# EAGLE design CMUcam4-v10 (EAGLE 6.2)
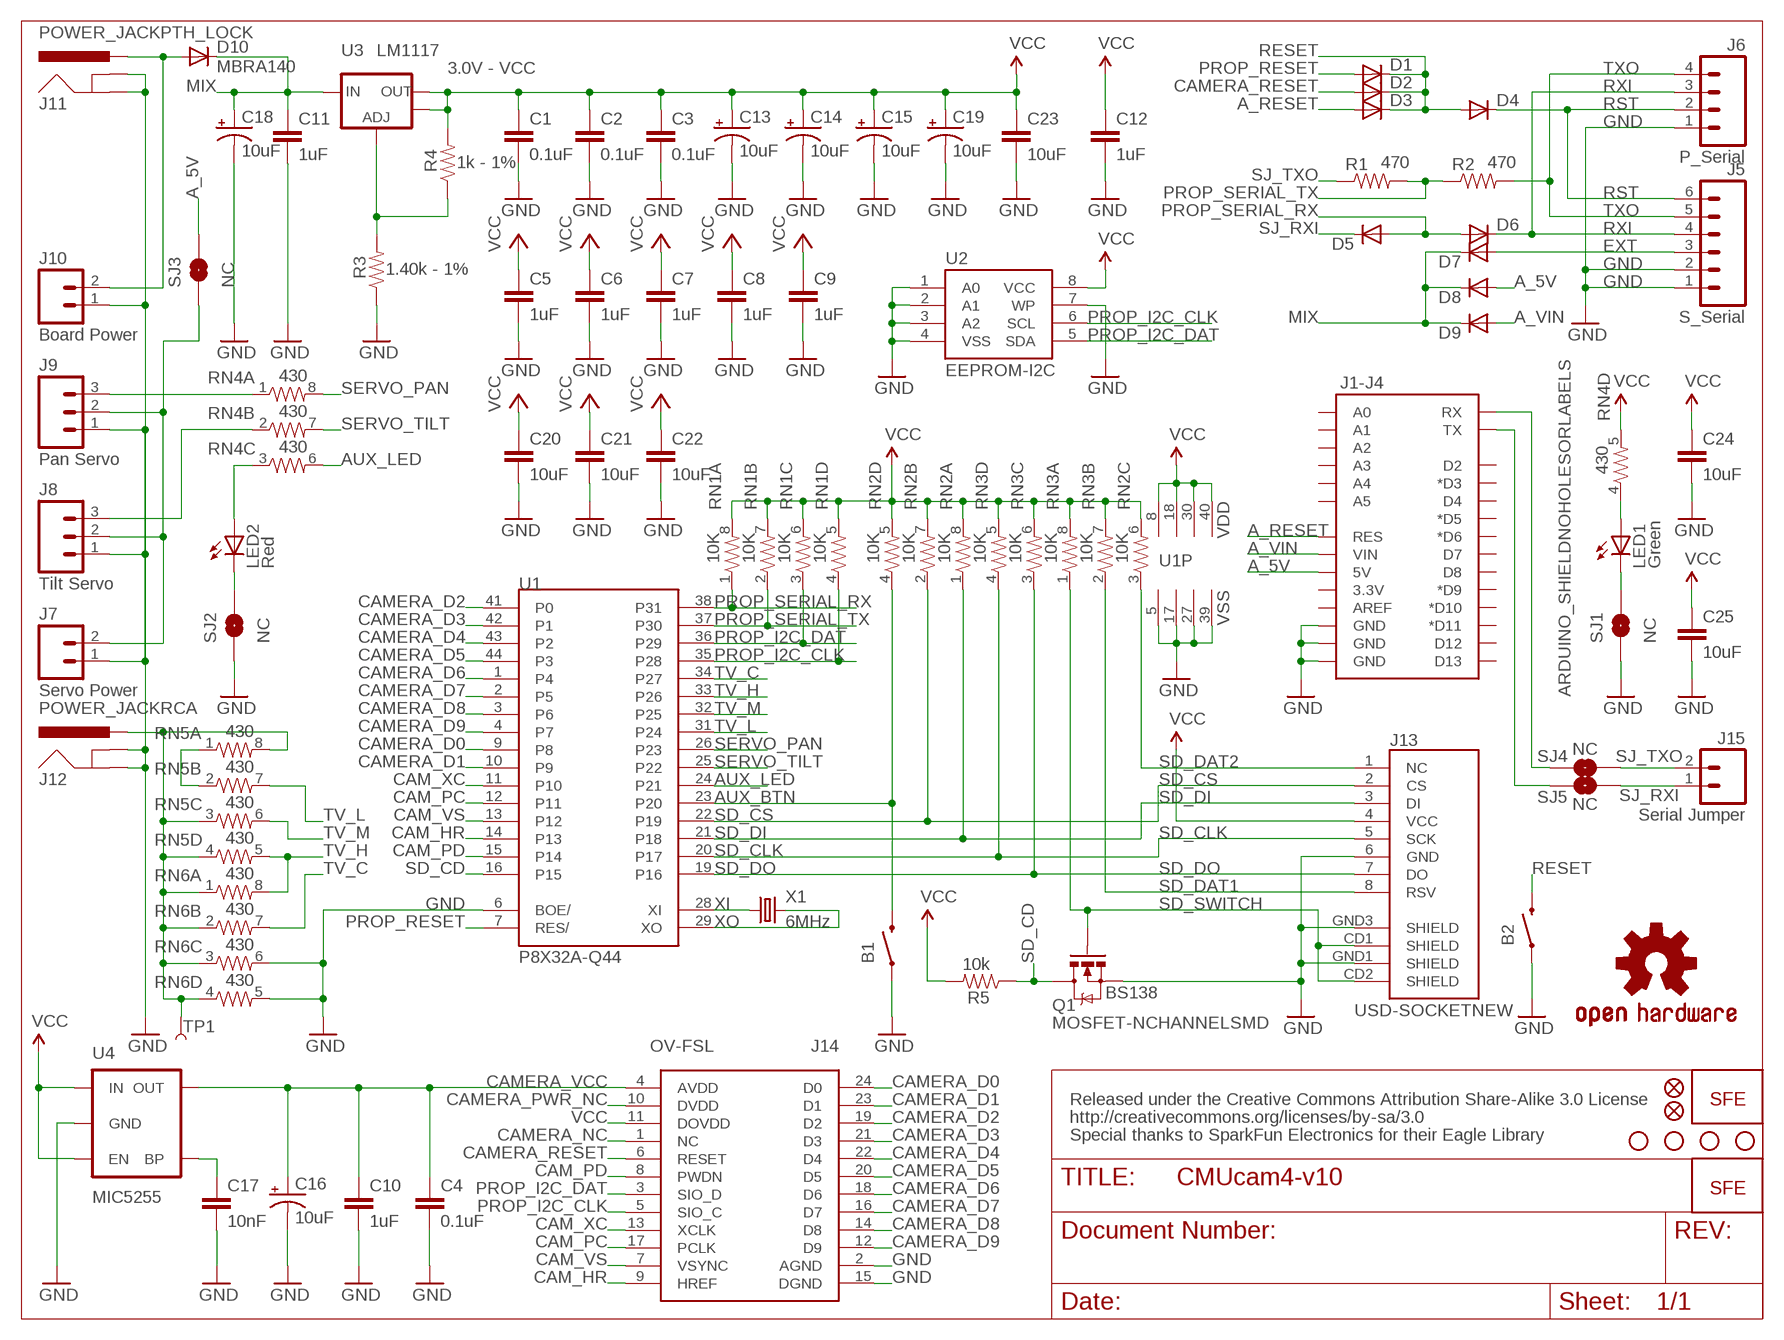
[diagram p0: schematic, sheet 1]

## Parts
B1  SWITCH-MOMENTARY-2SMD  [TACTILE_SWITCH_SMD]
B2  SWITCH-MOMENTARY-2SMD  [TACTILE_SWITCH_SMD]
C1  0.1uF  CAP0402-CAP  [0402-CAP]
C2  0.1uF  CAP0402-CAP  [0402-CAP]
C3  0.1uF  CAP0402-CAP  [0402-CAP]
C4  0.1uF  CAP0402-CAP  [0402-CAP]
C5  1uF  CAP0402-CAP  [0402-CAP]
C6  1uF  CAP0402-CAP  [0402-CAP]
C7  1uF  CAP0402-CAP  [0402-CAP]
C8  1uF  CAP0402-CAP  [0402-CAP]
C9  1uF  CAP0402-CAP  [0402-CAP]
C10  1uF  CAP0402-CAP  [0402-CAP]
C11  1uF  CAP0402-CAP  [0402-CAP]
C12  1uF  CAP0402-CAP  [0402-CAP]
C13  10uF  CAP_POL1206  [EIA3216]
C14  10uF  CAP_POL1206  [EIA3216]
C15  10uF  CAP_POL1206  [EIA3216]
C16  10uF  CAP_POL1206  [EIA3216]
C17  10nF  CAP0402-CAP  [0402-CAP]
C18  10uF  CAP_POL1206  [EIA3216]
C19  10uF  CAP_POL1206  [EIA3216]
C20  10uF  CAP0402-CAP  [0402-CAP]
C21  10uF  CAP0402-CAP  [0402-CAP]
C22  10uF  CAP0402-CAP  [0402-CAP]
C23  10uF  CAP0402-CAP  [0402-CAP]
C24  10uF  CAP0402-CAP  [0402-CAP]
C25  10uF  CAP0402-CAP  [0402-CAP]
D1  DIODESOD523  [SOD523]
D2  DIODESOD523  [SOD523]
D3  DIODESOD523  [SOD523]
D4  DIODESOD523  [SOD523]
D5  DIODESOD523  [SOD523]
D6  DIODESOD523  [SOD523]
D7  DIODESMA  [SMA-DIODE]
D8  DIODESMA  [SMA-DIODE]
D9  DIODESMA  [SMA-DIODE]
D10  MBRA140  DIODESMA  [SMA-DIODE]
J1-J4  ARDUINO_SHIELDNOHOLESORLABELS  [DUEMILANOVE_SHIELD_NOHOLES_NOLABELS]
J5  S_Serial  M06SIP  [1X06]
J6  P_Serial  M04PTH  [1X04]
J7  Servo Power  M02PTH  [1X02]
J8  Tilt Servo  M03PTH  [1X03]
J9  Pan Servo  M03PTH  [1X03]
J10  Board Power  M02PTH  [1X02]
J11  POWER_JACKPTH_LOCK  [POWER_JACK_PTH_LOCK]
J12  POWER_JACKRCA  [RCA]
J13  USD-SOCKETNEW  [MICRO-SD-SOCKET-PP]
J14  OV-FSL  [OV-FSL]
J15  Serial Jumper  M02PTH  [1X02]
JP1  LOGO-SFENEW  [SFE-NEW-WEBLOGO]
JP2  LOGO-SFESK  [SFE-LOGO-FLAME]
JP3  FIDUCIALUFIDUCIAL  [MICRO-FIDUCIAL]
JP4  FIDUCIALUFIDUCIAL  [MICRO-FIDUCIAL]
LED1  Green  LED0603  [LED-0603]
LED2  Red  LED0603  [LED-0603]
Q1  MOSFET-NCHANNELSMD  [SOT23-3]
R1  470  RESISTOR0402-RES  [0402-RES]
R2  470  RESISTOR0402-RES  [0402-RES]
R3  1.40k - 1%  RESISTOR0402-RES  [0402-RES]
R4  1k - 1%  RESISTOR0402-RES  [0402-RES]
R5  10k  RESISTOR0402-RES  [0402-RES]
RN1  10K  4R-N0603-ARV  [0603-ARV]
RN2  10K  4R-N0603-ARV  [0603-ARV]
RN3  10K  4R-N0603-ARV  [0603-ARV]
RN4  430  4R-N0603-ARV  [0603-ARV]
RN5  430  4R-N0603-ARV  [0603-ARV]
RN6  430  4R-N0603-ARV  [0603-ARV]
SJ1  NC  SOLDERJUMPERTRACE  [SJ_2S-TRACE]
SJ2  NC  SOLDERJUMPERTRACE  [SJ_2S-TRACE]
SJ3  NC  SOLDERJUMPERNO  [SJ_2S-NO]
SJ4  NC  SOLDERJUMPERTRACE  [SJ_2S-TRACE]
SJ5  NC  SOLDERJUMPERTRACE  [SJ_2S-TRACE]
STD1  STAND-OFF  [STAND-OFF]
STD2  STAND-OFF  [STAND-OFF]
STD3  STAND-OFF  [STAND-OFF]
STD4  STAND-OFF  [STAND-OFF]
TP1  TEST-POINT3  [PAD.03X.03]
U1  P8X32A-Q44  [P8X32A-Q44]
U2  EEPROM-I2C  [SO08-EIAJ]
U3  LM1117  V_REG_LM1117SOT223  [SOT223]
U4  MIC5255  V_REG_LDOSMD  [SOT23-5]
U$1  OSHW-LOGOM  [OSHW-LOGO-M]
X1  6MHz  CRYSTALHC49UP  [HC49UP]

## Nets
A_5V: D8.A J1-J4.5V SJ3.2
A_RESET: D3.A J1-J4.RES
A_VIN: D9.A J1-J4.VIN
ADJUST: R3.2 R4.1 U3.1(ADJ)
AUX_BTN: B1.3 RN2.4 U1.23(P20)
AUX_LED: RN4.6 U1.24(P21)
BYP: C17.1 U4.4(BP)
CAM_HR: J14.9(HREF) U1.14(P13)
CAM_PC: J14.17(PCLK) U1.12(P11)
CAM_PD: J14.8(PWDN) U1.15(P14)
CAM_VS: J14.7(VSYNC) U1.13(P12)
CAM_XC: J14.13(XCLK) U1.11(P10)
CAMERA_D0: J14.24(D0) U1.9(P8)
CAMERA_D1: J14.23(D1) U1.10(P9)
CAMERA_D2: J14.19(D2) U1.41(P0)
CAMERA_D3: J14.21(D3) U1.42(P1)
CAMERA_D4: J14.22(D4) U1.43(P2)
CAMERA_D5: J14.20(D5) U1.44(P3)
CAMERA_D6: J14.18(D6) U1.1(P4)
CAMERA_D7: J14.16(D7) U1.2(P5)
CAMERA_D8: J14.14(D8) U1.3(P6)
CAMERA_D9: J14.12(D9) U1.4(P7)
CAMERA_NC: J14.1(NC)
CAMERA_PWR_NC: J14.10(DVDD)
CAMERA_RESET: D2.A J14.6(RESET)
CAMERA_VCC: C4.1 C10.1 C16.A(+) J14.4(AVDD) U4.5(OUT)
D0_TXO: J1-J4.RX SJ4.1
D1_RXI: J1-J4.TX SJ5.1
EXT: D7.A J5.3
GND [vcc]: B1.1 B2.1 C1.2 C2.2 C3.2 C4.2 C5.2 C6.2 C7.2 C8.2 C9.2 C10.2 C11.2 C12.2 C13.C(-) C14.C(-) C15.C(-) C16.C(-) C17.2 C18.C(-) C19.C(-) C20.2 C21.2 C22.2 C23.2 C24.2 C25.2 J1-J4.GND@0(GND) J1-J4.GND@1(GND) J1-J4.GND@2(GND) J5.1 J5.2 J6.1 J7.1 J8.1 J9.1 J10.1 J11.GND J11.GNDBREAK J12.BARREL(GND) J12.SPRING(GNDBREAK) J13.6(GND) J13.GND1(SHIELD) J13.GND3(SHIELD) J14.2(AGND) J14.15(DGND) Q1.2(S) R3.1 RN6.5 RN6.6 SJ1.1 SJ2.1 U1.5(VSS) U1.6(BOE/) U1.17(VSS) U1.27(VSS) U1.39(VSS) U2.1(A0) U2.2(A1) U2.3(A2) U2.4(VSS) U2.7(WP) U4.2(GND)
GREEN_BRIDGE: LED1.C SJ1.2
GREEN_CTRL: LED1.A RN4.4
MIX: C11.1 C18.A(+) D7.C D8.C D9.C D10.C U3.3(IN)
PROP_I2C_CLK: J14.5(SIO_C) RN1.4 U1.35(P28) U2.6(SCL)
PROP_I2C_DAT: J14.3(SIO_D) RN1.3 U1.36(P29) U2.5(SDA)
PROP_RESET: D1.A U1.7(RES/)
PROP_SERIAL_RX: D5.A D6.A RN1.1 U1.38(P31)
PROP_SERIAL_TX: R1.2 R2.1 RN1.2 U1.37(P30)
RED_BRIDGE: LED2.C SJ2.2
RED_CTRL: LED2.A RN4.3
RESET: B2.3 D1.C D2.C D3.C D4.A
RST: D4.C J5.6 J6.2
RXI: D6.C J5.4 J6.3
SD_CD: Q1.3(D) R5.1 U1.16(P15)
SD_CLK: J13.5(SCK) RN3.4 U1.20(P17)
SD_CS: J13.2(CS) RN2.2 U1.22(P19)
SD_DAT1: J13.8(RSV) RN3.2
SD_DAT2: J13.1(NC) RN2.3
SD_DI: J13.3(DI) RN2.1 U1.21(P18)
SD_DO: J13.7(DO) RN3.3 U1.19(P16)
SD_SWITCH: J13.CD1(SHIELD) J13.CD2(SHIELD) Q1.1(G) RN3.1
SERVO_PAN: RN4.8 U1.26(P23)
SERVO_PAN_IO: J9.3 RN4.1
SERVO_PWR: J7.2 J8.2 J9.2 SJ3.1
SERVO_TILT: RN4.7 U1.25(P22)
SERVO_TILT_IO: J8.3 RN4.2
SJ_RXI: D5.C J15.1 SJ5.2
SJ_TXO: J15.2 R1.1 SJ4.2
SYSTEM_VIN: D10.A J10.2 J11.PWR
TV: J12.BREAK(PWR) RN5.3 RN5.4 RN5.8 RN6.1 RN6.2 RN6.3 RN6.4 TP1.P$1
TV_C: RN6.7 U1.34(P27)
TV_H: RN5.5 RN6.8 U1.33(P26)
TV_L: RN5.7 U1.31(P24)
TV_M: RN5.6 U1.32(P25)
TV_R: RN5.1 RN5.2
TXO: J5.5 J6.4 R2.2
VCC: C1.1 C2.1 C3.1 C5.1 C6.1 C7.1 C8.1 C9.1 C12.1 C13.A(+) C14.A(+) C15.A(+) C19.A(+) C20.1 C21.1 C22.1 C23.1 C24.1 C25.1 J13.4(VCC) J14.11(DOVDD) R4.2 R5.2 RN1.5 RN1.6 RN1.7 RN1.8 RN2.5 RN2.6 RN2.7 RN2.8 RN3.5 RN3.6 RN3.7 RN3.8 RN4.5 U1.8(VDD) U1.18(VDD) U1.30(VDD) U1.40(VDD) U2.8(VCC) U3.2(OUT) U3.4(OUT) U4.1(IN) U4.3(EN)
XI: U1.28(XI) X1.1
XO: U1.29(XO) X1.2
Unconnected: J1-J4.3.3V J1-J4.A0 J1-J4.A1 J1-J4.A2 J1-J4.A3 J1-J4.A4 J1-J4.A5 J1-J4.AREF J1-J4.D2 J1-J4.D3(*D3) J1-J4.D4 J1-J4.D5(*D5) J1-J4.D6(*D6) J1-J4.D7 J1-J4.D8 J1-J4.D9(*D9) J1-J4.D10(*D10) J1-J4.D11(*D11) J1-J4.D12 J1-J4.D13

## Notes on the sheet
- 3.0V - VCC
- BS138
- Released under the Creative Commons Attribution Share-Alike 3.0 License
- http://creativecommons.org/licenses/by-sa/3.0
- Special thanks to SparkFun Electronics for their Eagle Library

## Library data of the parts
B1 B2 = SparkFun:SWITCH-MOMENTARY-2
C1-C12 C17 C20-C25 = SparkFun:CAP: Capacitor
C13-C16 C18 C19 = SparkFun:CAP_POL: Capacitor Polarized
D1-D6 = SparkFun-DiscreteSemi:DIODE: Diode
D7-D10 = SparkFun:DIODE: Diode
J1-J4 = SparkFun:ARDUINO_SHIELD
J5 = SparkFun:M06: Header 6 Standard 6-pin 0.1" header. Use with straight break away headers (SKU : PRT-00116), right angle break away headers (PRT-00553), swiss pins (PRT-00743), machine pins (PRT-00117), and female headers (PRT-00115). Molex polarized connector foot print use with SKU : PRT-08094 with associated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
J6 = SparkFun:M04: Header 4 Standard 4-pin 0.1" header. Use with straight break away headers (SKU : PRT-00116), right angle break away headers (PRT-00553), swiss pins (PRT-00743), machine pins (PRT-00117), and female headers (PRT-00115). Molex polarized connector foot print use with SKU : PRT-08231 with associated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
J7 J10 J15 = SparkFun:M02: Header 2
J8 J9 = SparkFun:M03: Header 3 Standard 3-pin 0.1" header. Use with straight break away headers (SKU : PRT-00116), right angle break away headers (PRT-00553), swiss pins (PRT-00743), machine pins (PRT-00117), and female headers (PRT-00115). Molex polarized connector foot print use with SKU : PRT-08232 with associated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
J11 J12 = SparkFun:POWER_JACK: Power Jack This is the standard 5.5mm barrel jack for power. The PTH is the most common, proven, reliable, footprint. All others are experimental. The Slot footprint only works if the mill layer is transmitted to the PCB fab house so be warned. Spark Fun Electronics SKU : PRT-00119. Mating wall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
J13 = SparkFun:USD-SOCKET: microSD Socket Push-push type uSD socket. Schematic element and footprint production proven. Spark Fun Electronics SKU : PRT-00127. tDoc lines correctly indicate media card edge positions when inserting (unlocked, locked, depressed).
J14 = ovt-breakout:OV-FSL
JP1 JP2 = SparkFun:LOGO-SFE: Spark Fun Electronics PCB Logo
JP3 JP4 = SparkFun:FIDUCIAL: Fiducial Alignment Points
LED1 LED2 = SparkFun:LED: LEDs
Q1 = SparkFun:MOSFET-NCHANNEL
R1-R5 = SparkFun:RESISTOR: Resistor
RN1-RN6 = resistor-dil:4R-N: Array Chip Resistor Source: RS Component / Phycomp
SJ1-SJ5 = SparkFun:SOLDERJUMPER: Solder Jumper
STD1-STD4 = SparkFun:STAND-OFF: Stand Off
TP1 = SparkFun-Passives:TEST-POINT: Bare copper test points for troubleshooting or ICT
U1 = parallax-propeller:P8X32A-Q44
U2 = SparkFun:EEPROM-I2C
U3 = SparkFun:V_REG_LM1117: Voltage Regulator LM1117 Standard adjustable voltage regulator but in SMD form. Spark Fun Electronics SKU : COM-00595
U4 = SparkFun:V_REG_LDO: Voltage Regulator LDO Standard 150mA LDO voltage regulator in SOT-23 layout. Micrel part MIC5205. BP (by-pass) pin is used to lower output noise with 470pF cap.
U$1 = SparkFun:OSHW-LOGO: Open Source Hardware Logo This logo indicates the piece of hardware it is found on incorporates a OSHW license and/or adheres to the definition of open source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
X1 = crystal:CRYSTAL: CRYSTAL; OC_FARNELL: unknown; OC_NEWARK: unknown

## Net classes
0 default: width 0.203 mm
1 vcc: width 0.254 mm

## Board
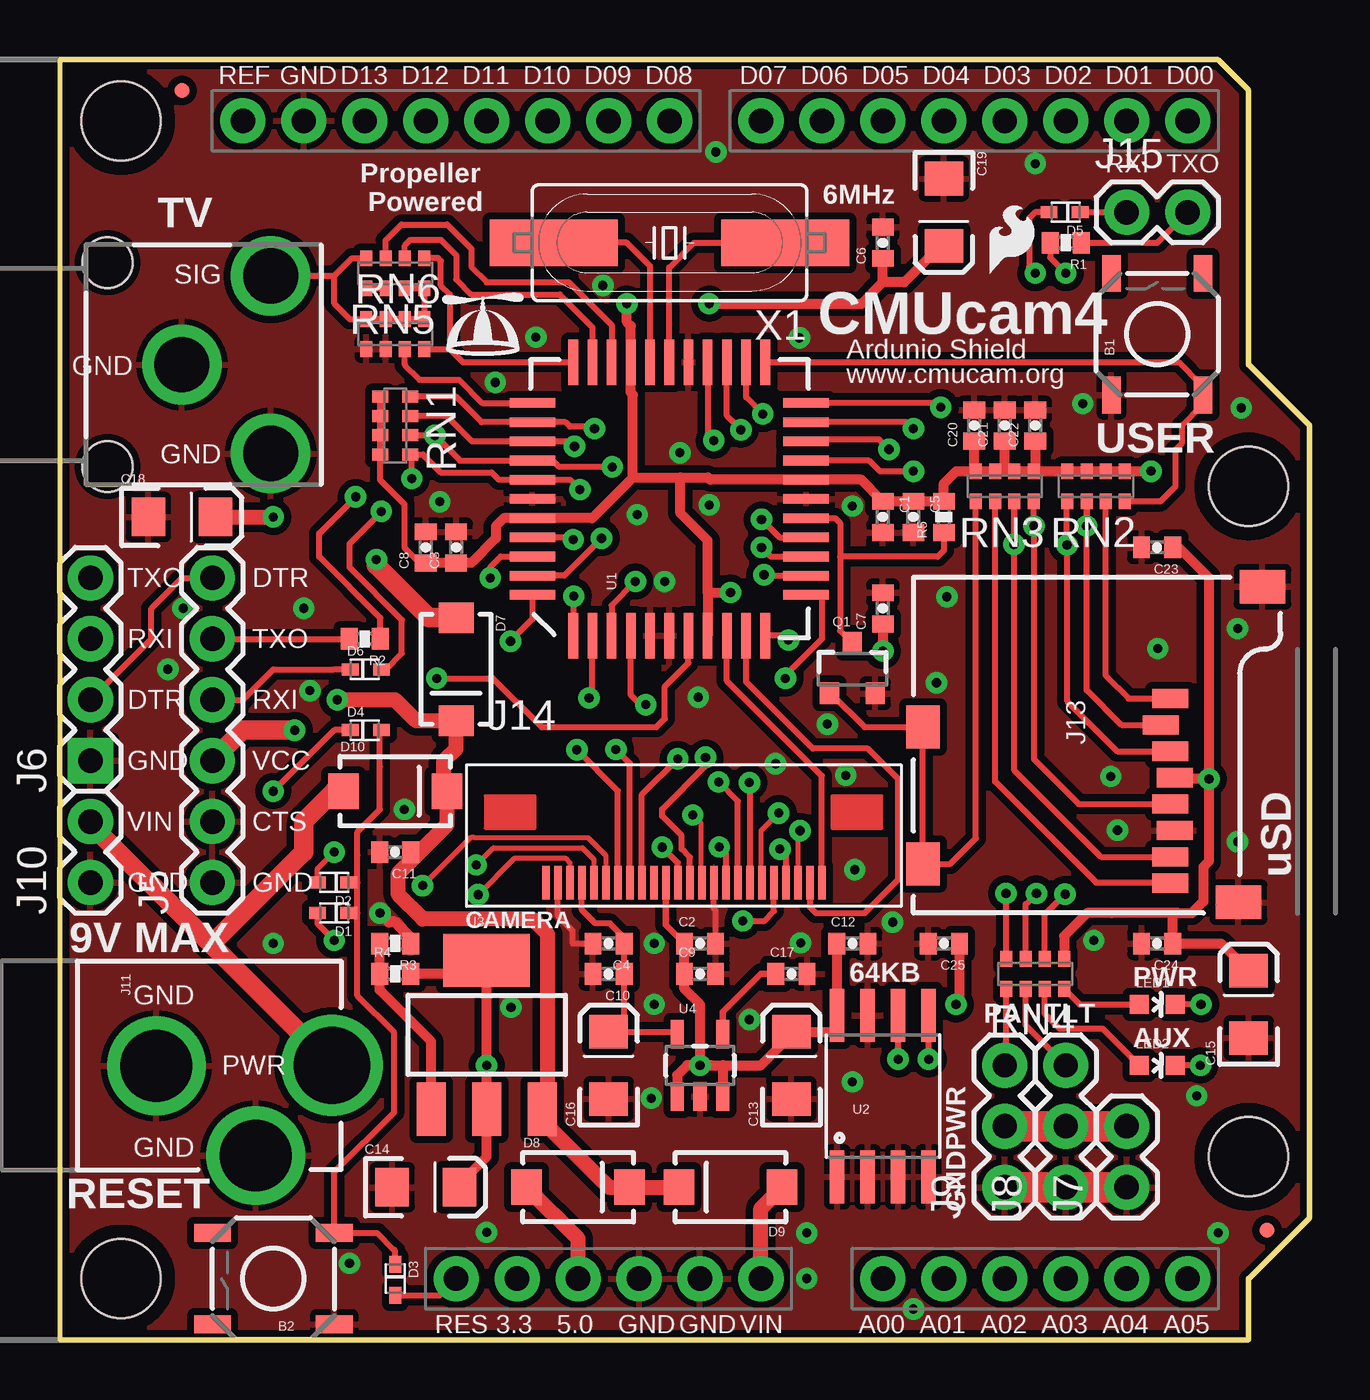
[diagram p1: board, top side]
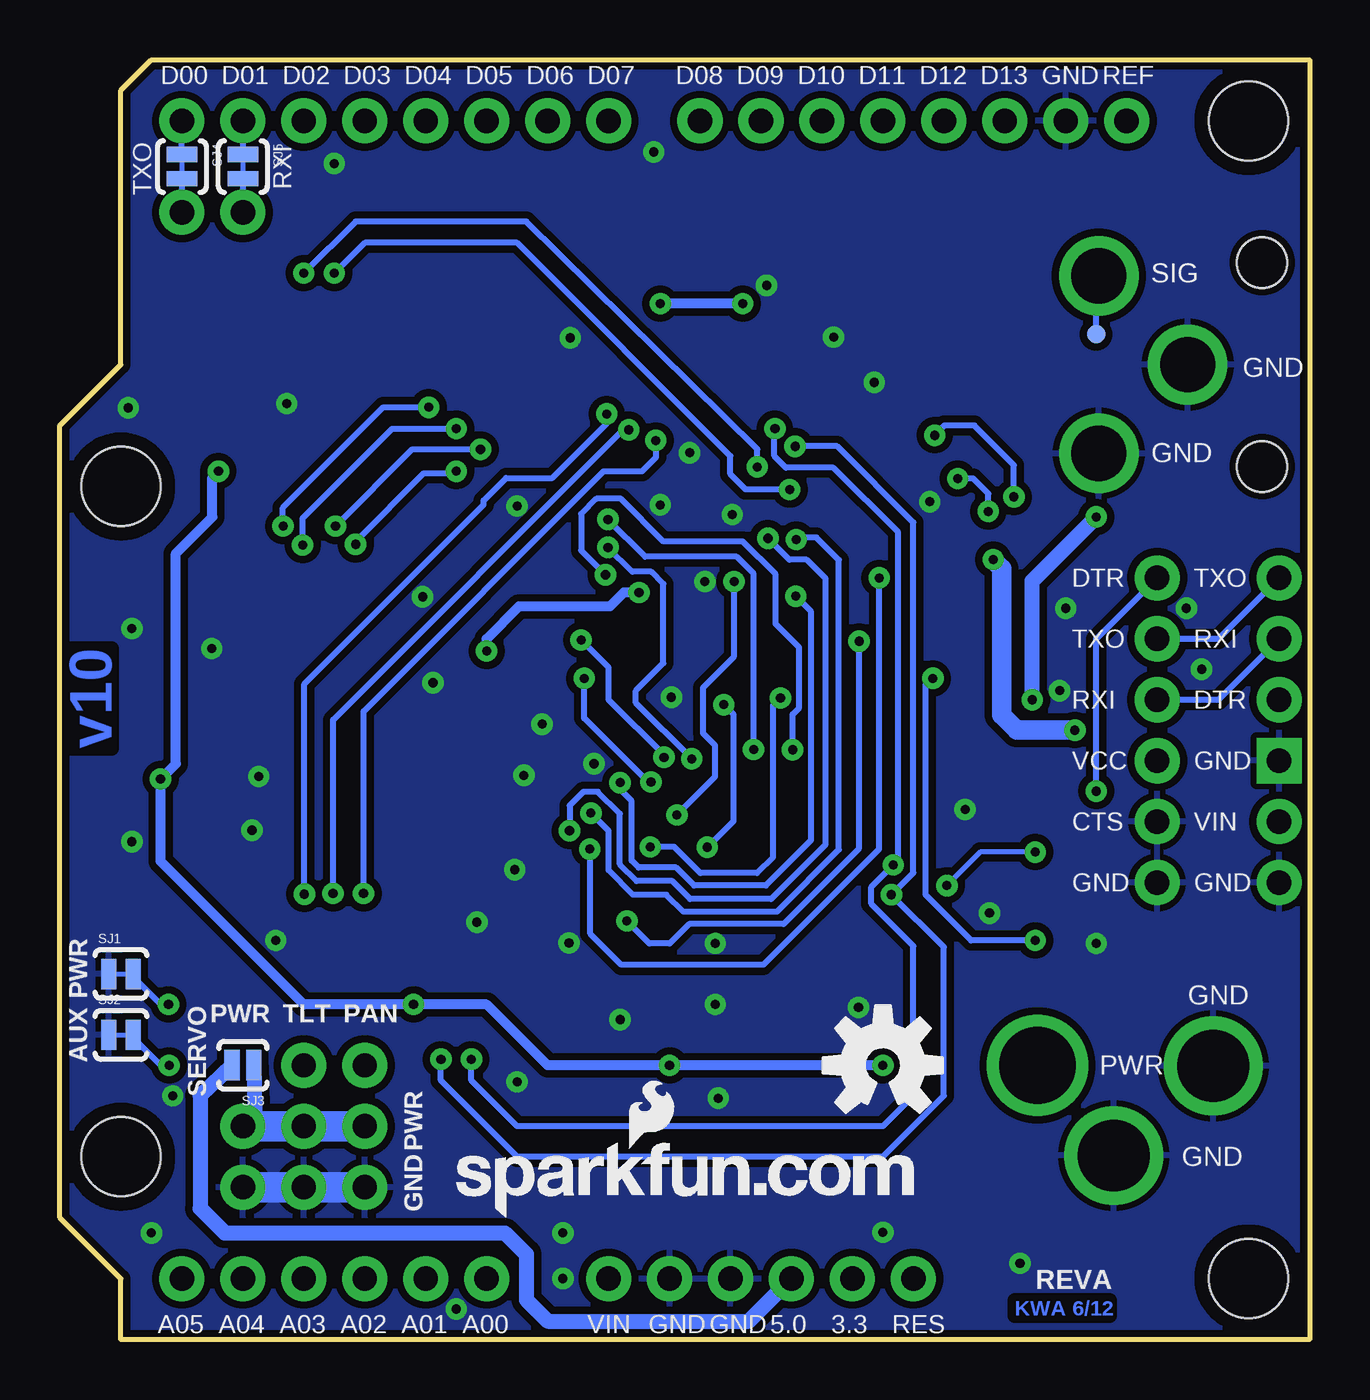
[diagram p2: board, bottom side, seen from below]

Size 52.07 x 53.34 mm. Coordinates in mm from the lower left corner, seen from the top.
Outline: 0,53.34 0,0 49.53,0 49.53,2.54 52.07,5.08 52.07,38.1 49.53,40.64 49.53,52.07 48.26,53.34 0,53.34
Copper layers (1*16): Top 0.035mm / dielectric 1.5mm / Bottom 0.035mm
Design rules: minimum track width 8mil, minimum drill 20mil, track to track 8mil, track to pad 8mil, pad to pad 8mil, via to via 8mil, smd to smd 8mil, copper to edge 10mil, drill to drill 8mil, minimum pad ring 12mil, minimum via ring 10mil, stop-mask expansion 4mil, vias tented up to drill 25mil, thermal gap 10mil
tRestrict: area 29.3,39.2 to 29.7,39.4; area 24.4,28.1 to 24.8,28.2; area 27.2,14.5 to 27.4,14.6; area 15.2,16.4 to 15.4,16.6; area 14.6,17 to 14.7,17.1; area 6.1,17.8 to 6.3,17.9; area 6.2,17.5 to 6.3,17.8

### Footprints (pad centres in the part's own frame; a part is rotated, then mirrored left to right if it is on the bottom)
TACTILE_SWITCH_SMD = smd 1.524 x 0.762: 1 -2.54,1.905; 2 2.54,1.905; 3 -2.54,-1.905; 4 2.54,-1.905
0402-CAP = smd 0.7 x 0.9: 1 -0.65,0; 2 0.65,0
EIA3216 = smd 1.4 x 1.6: A 1.4,0; C -1.4,0
SOD523 = smd 0.7 x 0.5: A 0.7,0; C -0.6,0
SMA-DIODE = smd 1.27 x 1.47: A -2.15,0; C 2.15,0
DUEMILANOVE_SHIELD_NOHOLES_NOLABELS = drill 1.016 pad 1.88: 3.3V 50.8,26.67; 5V 50.8,29.21; A0 50.8,41.91; A1 50.8,44.45; A2 50.8,46.99; A3 50.8,49.53; A4 50.8,52.07; A5 50.8,54.61; AREF 2.54,15.24; D2 2.54,49.53; D3 2.54,46.99; D4 2.54,44.45; D5 2.54,41.91; D6 2.54,39.37; D7 2.54,36.83; D8 2.54,33.02; D9 2.54,30.48; D10 2.54,27.94; D11 2.54,25.4; D12 2.54,22.86; D13 2.54,20.32; GND@0 50.8,31.75; GND@1 50.8,34.29; GND@2 2.54,17.78; RES 50.8,24.13; RX 2.54,54.61; TX 2.54,52.07; VIN 50.8,36.83
1X06 = drill 1.016 pad 1.88: 1 0,0; 2 2.54,0; 3 5.08,0; 4 7.62,0; 5 10.16,0; 6 12.7,0
1X04 = drill 1.016 pad 1.88 square: 1 0,0 | drill 1.016 pad 1.88: 2 2.54,0; 3 5.08,0; 4 7.62,0
1X02 = drill 1.016 pad 1.88: 1 0,0; 2 2.54,0
1X03 = drill 1.016 pad 1.88: 1 0,0; 2 2.54,0; 3 5.08,0
POWER_JACK_PTH_LOCK = drill 2.997 pad 4.115: GND 0.025,6.557; GNDBREAK 3.762,10.7 | drill 3.2 pad 4.115: PWR 0,13.878
RCA = drill 2.3: BARREL 0,0; BREAK 3.7,3.7; SPRING 3.7,-3.7 | hole 2.1: -3.1,4.25; -3.1,-4.25
MICRO-SD-SOCKET-PP = smd 0.8 x 1.5: 1 -8.94,10.7; 2 -7.84,10.3; 3 -6.74,10.7; 4 -5.64,10.9; 5 -4.54,10.7; 6 -3.44,10.9; 7 -2.34,10.7; 8 -1.24,10.7 | smd 1.8 x 1.4: CD1 -2.05,0.4; CD2 -7.75,0.4 | smd 1.4 x 1.9: GND1 -13.6,14.55; GND3 -0.45,13.55
OV-FSL = smd 0.3 x 1.4: 1 -5.15,-2.54; 2 -4.65,-2.54; 3 -4.15,-2.54; 4 -3.65,-2.54; 5 -3.15,-2.54; 6 -2.65,-2.54; 7 -2.15,-2.54; 8 -1.65,-2.54; 9 -1.15,-2.54; 10 -0.65,-2.54; 11 -0.15,-2.54; 12 0.35,-2.54; 13 0.85,-2.54; 14 1.35,-2.54; 15 1.85,-2.54; 16 2.35,-2.54; 17 2.85,-2.54; 18 3.35,-2.54; 19 3.85,-2.54; 20 4.35,-2.54; 21 4.85,-2.54; 22 5.35,-2.54; 23 5.85,-2.54; 24 6.35,-2.54
MICRO-FIDUCIAL = smd 0.635 x 0.635: 1 0,0
LED-0603 = smd 0.8 x 0.8: A 0,-0.75; C 0,0.75
SOT23-3 = smd 0.8 x 0.9: 1 -0.95,-1; 2 0.95,-1; 3 0,1.1
0402-RES = smd 0.7 x 0.9: 1 -0.65,0; 2 0.65,0
0603-ARV = smd 0.5 x 0.65: 1 -1.2,-0.625; 2 -0.4,-0.625; 3 0.4,-0.625; 4 1.2,-0.625; 5 1.2,0.625; 6 0.4,0.625; 7 -0.4,0.625; 8 -1.2,0.625
SJ_2S-TRACE = smd 0.635 x 1.27: 1 -0.508,0; 2 0.508,0
SJ_2S-NO = smd 0.635 x 1.27: 1 -0.45,0; 2 0.45,0
STAND-OFF = hole 3.302: 0,0
PAD.03X.03 = smd 0.762 x 0.762: P$1 0,0
P8X32A-Q44 = smd 1.9 x 0.4: 1 -5.713,4.013; 2 -5.713,3.212; 3 -5.713,2.413; 4 -5.713,1.613; 5 -5.713,0.812; 6 -5.713,0.013; 7 -5.713,-0.787; 8 -5.713,-1.587; 9 -5.713,-2.388; 10 -5.713,-3.188; 11 -5.713,-3.987; 23 5.688,-3.987; 24 5.688,-3.188; 25 5.688,-2.388; 26 5.688,-1.587; 27 5.688,-0.787; 28 5.688,0.013; 29 5.688,0.812; 30 5.688,1.613; 31 5.688,2.413; 32 5.688,3.212; 33 5.688,4.013 | smd 0.4 x 1.9: 12 -4.013,-5.688; 13 -3.212,-5.688; 14 -2.413,-5.688; 15 -1.613,-5.688; 16 -0.812,-5.688; 17 -0.013,-5.688; 18 0.787,-5.688; 19 1.587,-5.688; 20 2.388,-5.688; 21 3.188,-5.688; 22 3.987,-5.688; 34 3.987,5.713; 35 3.188,5.713; 36 2.388,5.713; 37 1.587,5.713; 38 0.787,5.713; 39 -0.013,5.713; 40 -0.812,5.713; 41 -1.613,5.713; 42 -2.413,5.713; 43 -3.212,5.713; 44 -4.013,5.713
SO08-EIAJ = smd 0.61 x 2.21: 1 -1.905,-3.378; 2 -0.635,-3.378; 3 0.635,-3.378; 4 1.905,-3.378; 5 1.905,3.353; 6 0.635,3.353; 7 -0.635,3.353; 8 -1.905,3.353
SOT223 = smd 1.219 x 2.235: 1 -2.311,-3.099; 2 0,-3.099; 3 2.311,-3.099 | smd 3.6 x 2.2: 4 0,3.099
SOT23-5 = smd 0.55 x 1.2: 1 -0.95,-1.3; 2 0,-1.3; 3 0.95,-1.3; 4 0.95,1.3; 5 -0.95,1.3
HC49UP = smd 5.334 x 1.93: 1 -4.826,0; 2 4.826,0

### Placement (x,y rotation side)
B1  45.72,41.91 90 top
B2  8.89,2.54 180 top
C1  34.29,34.29 270 top
C2  26.67,16.51 0 top
C3  16.51,33.02 90 top
C4  22.86,16.51 180 top
C5  35.56,34.29 270 top
C6  34.29,45.72 90 top
C7  34.29,30.48 90 top
C8  15.24,33.02 90 top
C9  26.67,15.24 0 top
C10  22.86,15.24 180 top
C11  13.97,20.32 180 top
C12  33.02,16.51 0 top
C13  30.48,11.43 90 top
C14  15.24,6.35 0 top
C15  49.53,13.97 90 top
C16  22.86,11.43 90 top
C17  30.48,15.24 0 top
C18  5.08,34.29 0 top
C19  36.83,46.99 270 top
C20  38.1,38.1 90 top
C21  39.37,38.1 90 top
C22  40.64,38.1 90 top
C23  45.72,33.02 180 top
C24  45.72,16.51 180 top
C25  36.83,16.51 180 top
D1  11.43,17.78 180 top
D2  11.43,19.05 180 top
D3  13.97,2.54 270 top
D4  12.7,25.4 0 top
D5  41.91,46.99 180 top
D6  12.7,27.94 0 top
D7  16.51,27.94 270 top
D8  21.59,6.35 0 top
D9  27.94,6.35 180 top
D10  13.97,22.86 0 top
J1-J4  -7.62,53.34 270 top
J5  6.35,19.05 90 top
J6  1.27,24.13 90 top
J7  44.45,6.35 90 top
J8  41.91,6.35 90 top
J9  39.37,6.35 90 top
J10  1.27,19.05 90 top
J11  -2.54,11.43 270 top
J12  5.08,40.64 0 top
J13  35.56,17.78 270 top
J14  25.4,21.59 0 top
J15  44.45,46.99 0 top
JP1  35.56,5.08 0 bottom
JP2  38.73,44.45 0 top
JP3  5.08,52.07 0 top
JP4  50.29,4.57 0 top
LED1  45.72,13.97 270 top
LED2  45.72,11.43 270 top
Q1  33.02,27.94 0 top
R1  41.91,45.72 180 top
R2  12.7,29.21 180 top
R3  13.97,16.51 180 top
R4  13.97,15.24 0 top
R5  36.83,34.29 90 top
RN1  13.97,38.1 90 top
RN2  43.18,35.56 0 top
RN3  39.37,35.56 0 top
RN4  40.64,15.24 0 top
RN5  13.97,44.45 0 top
RN6  13.97,41.91 180 top
SJ1  49.53,15.24 0 bottom
SJ2  49.53,12.7 0 bottom
SJ3  44.45,11.43 180 bottom
SJ4  46.99,48.9 270 bottom
SJ5  44.45,48.9 270 bottom
STD1  2.54,50.8 0 top
STD2  49.53,7.62 0 top
STD3  49.53,35.56 0 top
STD4  2.54,2.54 0 top
TP1  8.89,41.91 0 bottom
U1  25.4,35.05 90 top
U2  34.29,10.16 0 top
U3  17.78,12.7 0 top
U4  26.67,11.43 0 top
U$1  17.78,11.43 0 bottom
X1  25.4,45.72 180 top

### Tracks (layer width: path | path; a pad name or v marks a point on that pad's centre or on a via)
A_5V
  Top 0.635: J1-J4.5V 21.59,4.2 D8.A
  Bottom 0.635: SJ3.2 46.23,10.16 46.23,5.46 45.21,4.45 33.53,4.45 32.64,3.56 32.64,1.65 31.75,0.76 23.37,0.76 J1-J4.5V
A_RESET
  Top 0.254: D3.A 15.81,1.84 J1-J4.RES
A_VIN
  Top 0.635: J1-J4.VIN 29.21,5.47 D9.A
ADJUST
  Top 0.406: R3.2 R4.1 13.32,14.57 15.47,12.42 U3.1
AUX_BTN
  Top 0.254: RN2.4 45.86,34.94 46.48,35.56 46.48,37.08 46.74,37.34 46.74,38.1 47.62,38.99 B1.3 47.5,39.5 47.5,39.88 46.64,40.74 U1.23
AUX_LED  (via drill 0.38)
  Top 0.254: U1.24 28.59,39.28 v29.29,38.58 | RN4.6 41.04,17.72 v41.88,18.57
  Bottom 0.254: v29.29,38.58 29.29,38.18 31.55,35.92 33.48,35.92 34.42,34.98 34.42,34.8 41.88,27.33 v41.88,18.57
BYP
  Top 0.279: U4.4 27.62,13.65 29.21,15.24 C17.1
CAM_HR  (via drill 0.38)
  Top 0.254: U1.14 29.62,32.64 v29.23,33.02 | J14.9 24.25,22.71 v25.74,24.21
  Bottom 0.254: v25.74,24.21 v25.74,24.22 28.07,26.54 28.07,27.05 26.92,28.19 26.92,31.5 27.43,32 28.22,32 v29.23,33.02
CAM_PC  (via drill 0.38)
  Top 0.254: J14.17 28.25,22.44 v27.45,23.24 | U1.12 31.75,31.04 31.75,29.21 30.23,27.69 v30.23,27.56
  Bottom 0.254: v27.45,23.24 27.56,23.24 30.23,25.91 v30.23,27.56
CAM_PD  (via drill 0.38)
  Top 0.254: U1.15 29.98,33.44 v29.23,34.19 | J14.8 23.75,24.02 v23.16,24.6
  Bottom 0.254: v23.16,24.6 23.16,31.93 23.88,32.64 27.69,32.64 v29.23,34.19
CAM_VS  (via drill 0.38)
  Top 0.254: U1.13 29.38,31.84 v29.34,31.88 | J14.7 23.25,22.88 v21.54,24.59
  Bottom 0.254: v21.54,24.59 21.54,26.06 21.27,26.33 21.27,28.85 22.25,29.83 22.25,31.9 23.62,33.27 26.92,33.27 28.7,35.05 29.72,35.05 30.35,34.42 30.35,32.89 v29.34,31.88
CAM_XC  (via drill 0.38)
  Top 0.254: J14.13 26.25,20.11 25.91,20.45 25.91,21.01 25.09,21.82 25.09,22.1 26.9,23.9 v26.9,24.27 | U1.11 30.17,29.34 v30.35,29.16
  Bottom 0.254: v26.9,24.27 26.9,24.36 29.21,26.67 29.21,28.02 v30.35,29.16
CAMERA_D0
  Top 0.254: U1.9 27.79,27.46 31.75,23.5 J14.24
CAMERA_D1
  Top 0.254: J14.23 31.25,18.03 31.5,17.78 33.53,17.78 34.92,19.18 34.92,23.37 33.66,24.64 31.37,24.64 28.59,27.42 U1.10
CAMERA_D2  (via drill 0.38)
  Top 0.203: J14.19 29.21,19.1 29.21,21.21 v29.95,21.95
  Top 0.254: U1.41 21.3,33.44 v21.39,33.35
  Bottom 0.254: v29.95,21.95 29.21,21.21 29.21,19.56 28.19,18.54 26.8,18.54 26.09,17.83 22.2,17.83 19.61,20.42 19.61,32.5 20.55,33.44 21.3,33.44 v21.39,33.35
CAMERA_D3  (via drill 0.38)
  Top 0.254: J14.21 30.25,20.19 v30,20.45 | v17.93,31.75 17.93,32.21 18.36,32.64 U1.42
  Bottom 0.254: v17.93,31.75 17.93,20.45 22.76,15.62 28.68,15.62 29.97,16.92 29.97,20.42 v30,20.45
CAMERA_D4  (via drill 0.38)
  Top 0.203: J14.22 30.75,20.95 30.75,21.12 v30.84,21.21
  Top 0.254: U1.43 21.01,31.84 v22.57,33.4
  Bottom 0.254: v30.84,21.21 30.84,22.26 30.26,22.84 29.65,22.84 28.74,21.92 28.74,19.81 28.04,19.11 26.56,19.11 25.81,18.36 22.44,18.36 20.17,20.64 20.17,31.73 20.95,32.51 21.68,32.51 v22.57,33.4
CAMERA_D5  (via drill 0.38)
  Top 0.254: J14.20 29.75,17.86 29.34,17.45 v28.45,17.45 | 18.87,29.21 v18.77,29.11 19.69,30.02 U1.44
  Bottom 0.254: v18.77,29.11 18.77,20.47 21.92,17.32 25.86,17.32 26.67,16.51 27.51,16.51 v28.45,17.45
CAMERA_D6  (via drill 0.38)
  Top 0.254: J14.18 28.75,23.19 v28.73,23.22 | U1.1 21.39,30.96 v21.41,30.99
  Bottom 0.254: v28.73,23.22 28.73,22.92 28.25,22.44 28.25,19.96 27.95,19.67 26.39,19.67 25.64,18.92 22.66,18.92 20.77,20.82 20.77,30.34 v21.41,30.99
CAMERA_D7  (via drill 0.38)
  Top 0.254: J14.16 27.75,20.26 v27.47,20.54 | U1.2 22.19,26.89 v22.05,26.75
  Bottom 0.254: v27.47,20.54 26.48,20.54 25.39,19.44 23.02,19.44 22.35,20.12 22.35,26.44 v22.05,26.75
CAMERA_D8  (via drill 0.38)
  Top 0.203: J14.14 26.75,19.16 26.72,19.19 26.72,21.51 v26.36,21.87
  Top 0.254: 22.99,29.97 U1.3 22.99,30.61 v23.98,31.6
  Bottom 0.254: v23.98,31.6 23.98,28.47 25.27,27.18 25.27,25.27 24.77,24.77 24.77,23.47 v26.36,21.87
CAMERA_D9  (via drill 0.38)
  Top 0.254: J14.12 25.75,19.87 v25.09,20.52 | U1.4 23.79,26.86 24.18,26.47 v24.41,26.47
  Bottom 0.254: v25.09,20.52 24,21.61 24,26.06 v24.41,26.47
CAMERA_RESET  (via drill 0.38)
  Top 0.203: J14.6 22.75,20.18 22,20.93 17.27,20.93 17.12,20.93 v15.11,18.92 | D2.A 10.73,19.62 v11.43,20.32
  Bottom 0.203: v11.43,20.32 13.72,20.32 v15.11,18.92
CAMERA_VCC
  Top 0.254: U4.5 25.62,12.83 C16.A 23.51,13.48 C10.1 C4.1 23.51,16.75 22.91,17.35 22.3,17.35 21.75,17.9 J14.4
D0_TXO
  Bottom 0.254: SJ4.1 J1-J4.RX
D1_RXI
  Bottom 0.254: J1-J4.TX SJ5.1
EXT  (via drill 0.38)
  Top 0.813: v9.78,25.4 7.62,25.4 J5.3 | D7.A 15.38,30.09 13.18,32.28 v13.18,32.51
  Bottom 0.813: v13.18,32.51 13.21,32.51 12.83,32.13 12.83,26.04 12.19,25.4 v9.78,25.4
GND  (via drill 0.38)
  Top 0.254: J14.15 27.25,17.96 27.3,17.91 27.3,16.51 27.36,16.51 | J14.2 20.75,17.66 21.36,17.04 21.36,16.54 21.39,16.51 C4.2 | R3.1 14.62,16.75
  Top 0.457: 14.62,16.75 13.97,17.4 13.72,17.4 v13.34,17.78
  Top 1.27: J9.1 J7.1
  Bottom 1.27: J9.1 J7.1
  other vias: 33.02,34.75 14.35,22.1 44.07,21.23 36.96,30.96 36.53,27.38 32.74,23.52 24.77,16.51 25.2,31.6 24.77,13.97 26.59,26.77 24.05,34.39 25.83,36.97 15.82,34.92 30.86,16.54 24.64,10.06 31.98,25.65 4.5,27.94 43.79,23.47 45.75,28.8 49.07,29.64 40.64,49.02 19.83,41.78 49.23,38.84 33.02,10.74 34.7,17.4 27.33,49.5 10.16,30.48 8.89,16.51 18.14,39.9 30.81,41.76 33.12,19.58 42.62,39.01 22.62,43.94 27.06,34.79 18.8,13.84 28.73,13.34 17.78,4.47 29.82,24 10.41,27.05 43.08,16.64 5.13,30.48 49.07,20.75 31.11,4.45 12.06,3.17 35.56,1.27 48.26,4.45 47.37,10.16 31.11,2.54
  pour Top (isolate 0.305): 0,53.34 52.07,53.34 52.07,0 0,0
  pour Bottom (isolate 0.305): 0,53.34 52.07,53.34 52.07,0 0,0
GREEN_BRIDGE  (via drill 0.38)
  Top 0.254: v47.55,13.97 LED1.C
  Bottom 0.254: v47.55,13.97 47.88,13.97 49.02,15.11 SJ1.2
GREEN_CTRL
  Top 0.254: RN4.4 42.48,13.97 LED1.A
MIX  (via drill 0.38)
  Top 0.254: 16.51,23.25 D10.C 15.89,22.63
  Top 0.635: D9.C D8.C 22.86,6.35 20.32,8.89 20.32,9.37 U3.3 20.09,9.8 20.32,10.03 20.32,16.9 19.7,17.53 15.11,17.53 14.1,18.54 14.1,19.43 14.99,20.32 | D10.C 16,22.98 16,24.13 16.51,24.64 D7.C 14.85,25.79 13.97,26.67 v11.56,26.67 | 14.61,20.32 C11.1 14.99,20.32 | 14.99,20.32 16.13,21.46 16.13,22.35 15.88,22.61 | 15.88,22.61 16,22.61 | 15.89,22.63 15.89,22.62 15.88,22.61 | C18.A v8.89,34.29
  Bottom 0.635: v11.56,26.67 11.56,31.62 v8.89,34.29
PROP_I2C_CLK  (via drill 0.38)
  Top 0.203: v17.35,19.79 18.06,20.5 21.77,20.5 22.25,20.02 J14.5
  Top 0.254: RN1.4 16.51,39.3 17.57,38.24 U1.35 21.07,38.24 21.26,38.05 22.2,38.05 v22.28,37.97 | v34.92,11.68 U2.6
  Bottom 0.254: v34.92,11.68 34.92,10.79 33.02,8.89 17.78,8.89 16.51,10.16 16.51,16.41 18.26,18.16 18.26,18.87 v17.35,19.79 17.14,19.99 17.14,33.66 19.84,36.35 21.82,36.35 22.3,36.83 22.3,37.95 v22.28,37.97
PROP_I2C_DAT  (via drill 0.38)
  Top 0.203: v17.42,18.54 18.95,20.07 21.06,20.07 21.25,19.87 J14.3
  Top 0.254: RN1.3 16.11,38.5 17.17,37.44 U1.36 21.23,37.44 v21.44,37.24 | v36.2,11.68 U2.5
  Bottom 0.254: v36.2,11.68 36.2,10.79 33.02,7.62 17.78,7.62 15.24,10.16 15.24,16.36 v17.42,18.54 16.51,19.46 16.51,34.06 19.68,37.24 v21.44,37.24
PROP_RESET  (via drill 0.38)
  Top 0.254: U1.7 26.19,28.21 25.21,27.23 25.21,25.88 24.85,25.53 20.07,25.53 18.03,27.56 v15.7,27.56 | D1.A 10.73,17.34 v11.43,16.64
  Bottom 0.254: v11.43,16.64 14.1,16.64 16,18.54 16,27.3 15.75,27.56 v15.7,27.56
PROP_SERIAL_RX  (via drill 0.38)
  Top 0.203: 13.39,34.49 v13.39,34.52
  Top 0.254: v14.66,35.89 14.66,36.84 RN1.1 15.12,36.9 15.88,36.14 17.98,36.14 18.29,35.84 U1.38 21.26,35.84 v21.67,35.43 | 13.39,34.49 12.06,33.17 12.06,32.18 14.25,30 14.25,28.6 13.59,27.94 D6.A | D5.A 40.64,46.99 40.39,46.74 40.39,44.7 v40.64,44.45
  Bottom 0.254: v13.39,34.52 13.39,35.26 14.02,35.89 v14.66,35.89 | v21.67,35.43 23.5,35.43 24.13,36.07 24.13,36.83 33.02,45.72 39.37,45.72 v40.64,44.45
PROP_SERIAL_TX  (via drill 0.38)
  Top 0.203: 15.64,37.7 v15.63,37.7 v15.62,37.69
  Top 0.254: v23.01,36.37 22.99,36.4 20.78,36.4 20.54,36.64 U1.37 16.68,36.64 v15.62,37.69 RN1.2 | v12.32,35.13 10.79,33.6 10.79,32.64 13.35,30.08 R2.1 | R1.2 41.26,45.1 v41.91,44.45
  Bottom 0.254: v12.32,35.13 12.32,36.45 13.97,38.1 15.21,38.1 v15.62,37.69 | v23.01,36.37 23.01,37.11 32.64,46.61 39.75,46.61 v41.91,44.45
RED_BRIDGE  (via drill 0.38)
  Top 0.254: v47.52,11.43 LED2.C
  Bottom 0.254: SJ2.2 49.02,12.57 47.88,11.43 v47.52,11.43
RED_CTRL
  Top 0.254: RN4.3 41.04,13.57 41.66,12.95 43.45,12.95 LED2.A
RESET
  Top 0.254: 13.91,3.75 13.21,4.45 B2.3 11.43,6.99 13.92,9.47 13.92,12.8 12.39,14.33 12.39,17.78 | 13.91,3.75 13.97,3.69 | 12.39,17.78 12.39,19.05 | 12.39,19.05 12.39,20.19 | 12.39,20.19 12.39,21.16 13.34,22.1 13.34,23.88 13.34,25.27 13.46,25.4 D4.A | 12.39,20.19 12.39,20.2 | D1.C 12.39,17.78 | D2.C 12.39,19.05 | D3.C 13.97,3.69 | 13.97,3.69 13.91,3.75
RST  (via drill 0.38)
  Top 0.254: J6.2 3.81,29.21 3.81,30.48 5.08,31.75 J5.6 | D4.C 11.43,25.4 v8.89,22.86
  Bottom 0.254: v8.89,22.86 8.89,29.21 J5.6
RXI
  Top 0.254: J5.4 7.62,26.67 8.89,27.94 11.43,27.94 D6.C
  Bottom 0.254: J5.4 3.81,26.67 J6.3
SD_CD
  Top 0.254: U1.16 32.31,34.24 32.51,34.04 32.51,32.64 | 32.51,32.64 32.51,29.55 Q1.3 | R5.1 36.83,32.89 36.58,32.64 32.51,32.64
SD_CLK  (via drill 0.38)
  Top 0.254: J13.5 42.45,22.32 40.59,24.18 v40.59,33.91 40.57,33.93 RN3.4 | U1.20 31.67,37.44 31.75,37.52 34.14,37.52 v34.54,37.11
  Bottom 0.254: v34.54,37.11 37.39,37.11 v40.59,33.91
SD_CS  (via drill 0.38)
  Top 0.254: J13.2 44.23,25.62 42.78,27.07 RN2.2 v42.78,33.91 v42.77,33.91 | U1.22 36.53,39.04 v36.7,38.86
  Bottom 0.254: v42.77,33.91 v42.78,33.91 42.78,34.68 38.6,38.86 v36.7,38.86
SD_DAT1
  Top 0.254: RN3.2 38.97,23.26 43.18,19.05 46.23,19.05 J13.8
SD_DAT2
  Top 0.254: J13.1 44.53,26.72 43.58,27.67 RN2.3
SD_DI  (via drill 0.38)
  Top 0.254: J13.3 44.06,24.52 41.98,26.6 41.98,33.1 v41.96,33.12 41.96,34.92 RN2.1 | U1.21 35.29,38.24 v35.56,37.97
  Bottom 0.254: v41.96,33.12 41.96,34.24 38.23,37.97 v35.56,37.97
SD_DO  (via drill 0.38)
  Top 0.254: J13.7 43.38,20.12 39.77,23.73 RN3.3 39.77,33.17 v39.75,33.15 | U1.19 33.72,36.64 34.16,36.2 v35.56,36.2
  Bottom 0.254: v35.56,36.2 35.64,36.12 36.91,36.12 39.75,33.27 v39.75,33.15
SD_SWITCH
  Top 0.254: RN3.1 38.17,20.9 37.1,19.83 J13.CD1 J13.CD2 33.52,25.53 32.12,26.94 Q1.1
SERVO_PAN  (via drill 0.38)
  Top 0.254: RN4.8 39.44,18.57 v39.42,18.59 | U1.26 26.99,37.73 v27.24,37.48
  Bottom 0.254: v39.42,18.59 39.42,26.19 29.41,36.2 27.81,36.2 27.23,36.78 27.23,37.47 v27.24,37.48
SERVO_PAN_IO
  Top 0.254: RN4.1 39.44,11.5 J9.3
SERVO_PWR
  Top 1.27: J7.2 J8.2 J9.2
  Bottom 0.635: SJ3.1 43.94,8.89
  Bottom 1.27: J9.2 43.94,8.89 J7.2
SERVO_TILT  (via drill 0.38)
  Top 0.254: U1.25 27.79,38.51 v28.37,37.92 | RN4.7 40.24,18.14 v40.69,18.59
  Bottom 0.254: v40.69,18.59 40.69,25.83 28.6,37.92 v28.37,37.92
SERVO_TILT_IO
  Top 0.254: RN4.2 40.24,13.1 J8.3
SJ_RXI
  Top 0.254: D5.C J15.1
  Bottom 0.254: SJ5.2 J15.1
SJ_TXO
  Top 0.254: R1.1 45.72,45.72 J15.2
  Bottom 0.254: SJ4.2 J15.2
SYSTEM_VIN
  Top 0.254: J11.PWR 11.43,11.52
  Top 0.813: D10.A 11.43,22.86 10.16,21.59 10.16,20.32 6.3,16.46 | 10.16,12.61 J11.PWR 6.3,16.46 | J10.2 1.27,21.5 6.3,16.46
TV
  Top 0.203: 14.37,44.05 RN5.3 | RN5.8 12.77,44.89
  Top 0.254: RN5.3 RN5.4 RN6.1 RN6.2 RN6.3 RN6.4 12.07,42.53 11.43,43.18 11.43,44.34 | J12.BREAK 11.43,44.34 | 11.43,44.34 12.16,45.08 RN5.8
  Bottom 0.254: TP1.P$1 8.89,44.45 J12.BREAK
TV_C
  Top 0.254: RN6.7 14.37,40.62 14.99,40.01 16.64,40.01 17.6,39.04 U1.34
TV_H
  Top 0.254: 16.25,41.28 RN6.8 16.01,41.28 | 16.25,41.28 16.26,41.28 16.26,43.56 15.88,43.94 15.88,44.96 15.75,45.09 RN5.5 | U1.33 16.79,40.74 16.25,41.28
TV_L
  Top 0.254: U1.31 22.99,42.29 21.21,44.07 17.78,44.07 17.14,44.7 17.14,45.47 16.13,46.48 14.22,46.48 13.57,45.83 RN5.7
TV_M
  Top 0.254: U1.32 22.19,42.2 20.83,43.56 17.14,43.56 16.51,44.2 16.51,45.21 15.88,45.85 14.61,45.85 14.37,45.61 RN5.6
TV_R
  Top 0.254: RN5.1 RN5.2
TXO
  Top 0.254: J5.5 R2.2
  Bottom 0.254: J5.5 3.81,29.21 J6.4
VCC  (via drill 0.38)
  Top 0.203: C14.A 16.64,6.48
  Top 0.254: RN1.5 RN1.6 RN1.7 RN1.8 13.35,35.83 14.35,34.82 14.35,33.02 15,32.37 C8.1 | 23.88,39.37 23.79,39.46 | J13.4 47.01,23.42 47.07,23.37 | v45.47,36.2 45.46,36.19 | RN2.5 RN2.6 | RN2.5 44.45,36.2 44.44,36.19 RN2.5 | 32.38,16.52 C12.1
  Top 0.279: 43.81,17.78 43.8,17.77 | J14.11 25.25,17.28 C2.1
  Top 0.406: 23.79,39.46 U1.30 23.79,42.25 23.62,42.42 v23.62,43.18 | 23.88,35.94 23.88,39.37 | 23.88,35.94 22.17,34.24 U1.40 18.49,34.24 18.16,33.91 18.16,33.4 17.13,32.37 C3.1 C8.1 | RN3.8 RN3.7 39.37,36.19 | RN3.5 RN3.6 39.37,36.19 | RN3.5 RN2.8 RN2.7 RN2.6 RN2.5 45.46,36.19 | 16.64,6.48 17.78,7.62 U3.2 v17.78,11.43 17.78,15.24 | U4.1 25.72,11.01 26.14,11.43 v26.67,11.43 | v26.67,11.43 27.13,11.43 | v47.88,23.37 47.07,23.37 | RN4.5 41.84,16.82 42.8,17.78 43.81,17.78 46.35,17.78 | 46.35,17.78 46.62,17.78 47.17,17.78 47.65,18.26 47.65,19.71 47.88,19.94 v47.88,23.37 | v26.67,11.43 26.67,13.97 26.02,14.62 C9.1 C2.1 | 17.78,15.24 U3.4 | 17.78,15.24 R4.2 | 26.99,31.14 U1.8 | 32.38,16.52 U2.8 32.38,12.83 C13.A 30.48,12.7 29.21,11.43 27.62,11.43 | 49.03,15.87 C15.A 48.39,16.51 C24.1 46.37,17.77 46.35,17.78 | v26.67,11.43 27.62,11.43 | 27.62,11.43 U4.3 | 34.29,44.07 C6.1 34.4,44.96 | v27.05,43.18 33.4,43.18 34.29,44.07 | 26.99,31.14 v27.94,31.14 | 23.88,35.94 25.86,35.94 | 25.86,35.94 27,35.94 27.1,35.84 U1.18 33.39,35.84 C1.1 C5.1 R5.2 36.83,35.69 37.33,36.19 RN3.8 | 26.99,31.14 26.99,33.31 25.86,34.44 25.86,35.94 | C7.1 v34.29,28.7 | C19.A 36.7,45.59 35.18,44.07 34.29,44.07 | RN3.8 38.1,36.26 C20.1 | C22.1 40.64,36.19 RN3.5 | v47.88,23.37 47.88,31.76 46.62,33.02 C23.1 | 39.37,36.19 C21.1 | C25.1 37.48,14.11 v37.34,13.97
  Bottom 0.406: v17.78,11.43 v26.67,11.43 31.75,11.43 34.29,13.97 v37.34,13.97 41.91,13.97 47.88,19.94 v47.88,23.37 47.24,24 47.24,32.77 45.72,34.29 45.72,35.94 v45.47,36.2 | v23.62,43.18 v27.05,43.18 | v27.94,31.14 28.57,31.14 29.16,30.56 32.94,30.56 34.29,29.21 v34.29,28.7
XI
  Top 0.254: X1.1 26.42,45.72 25.39,44.69 U1.28
XO
  Top 0.254: X1.2 23.62,45.72 24.59,44.76 U1.29

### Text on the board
Bottom: v10 | KWA 6/12
tPlace: REF | GND | D13 | D12 | D11 | D10 | D09 | D08 | D07 | D06 | D05 | D04 | D03 | D02 | D01 | D00 | RXI | TXO | Propeller | Powered | 6MHz | TV | SIG | CMUcam4 | GND | Ardunio Shield | www.cmucam.org | USER | GND | TXO | DTR | RXI | TXO | DTR | RXI | GND | VCC | uSD | VIN | CTS | GND | GND | CAMERA | 9V MAX | 64KB | PWR | GND | PAN | TLT | AUX | PWR | GND | PWR | RESET | GND | RES | 3.3 | 5.0 | GND | GND | VIN | A00 | A01 | A02 | A03 | A04 | A05
bPlace: REF | GND | D13 | D12 | D11 | D10 | D09 | D08 | D07 | D06 | D05 | D04 | D03 | D02 | D01 | D00 | RXI | TXO | SIG | GND | GND | TXO | DTR | RXI | TXO | DTR | RXI | GND | VCC | VIN | CTS | GND | GND | GND | PWR | SERVO | PWR | AUX | PAN | TLT | PWR | PWR | GND | GND | REVA | RES | 3.3 | 5.0 | GND | GND | VIN | A00 | A01 | A02 | A03 | A04 | A05
tDocu: Released under the Creative Commons Attribution Share-Alike 3.0 License | http://creativecommons.org/licenses/by-sa/3.0 | Special thanks to SparkFun Electronics for their Eagle Library

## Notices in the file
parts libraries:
SparkFun-DiscreteSemi: Licensing: CC v3.0 Share-Alike You are welcome to use this library for commercial purposes.
